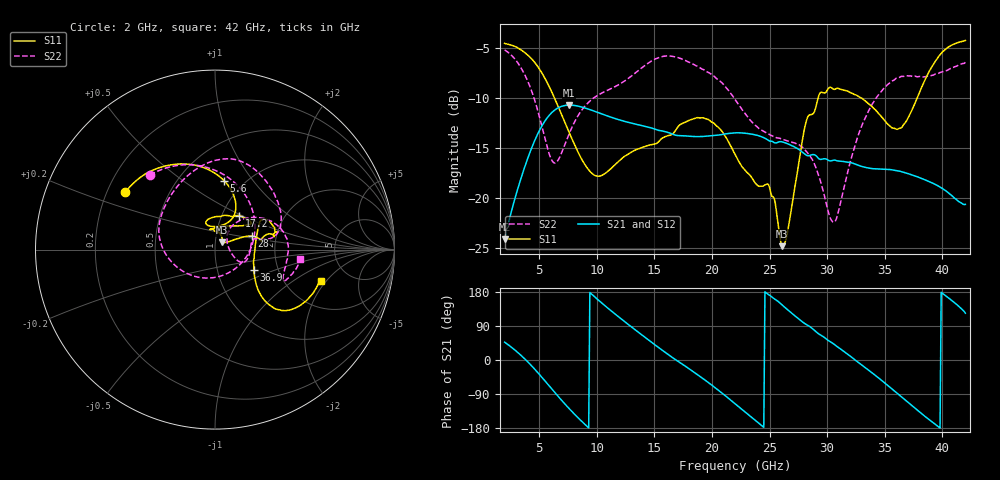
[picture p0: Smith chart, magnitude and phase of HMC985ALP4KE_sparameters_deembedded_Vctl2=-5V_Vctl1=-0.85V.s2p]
!s2p File: Measurements: S11, S21, S12, S22
# GHz S dB R 50.0
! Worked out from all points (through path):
!   401 points, 2 GHz to 42 GHz, reference 50 ohm
!   highest |S21| = -10.71 dB at 7.6 GHz (marker M1); lowest = -24.2 dB at 2 GHz (marker M2)
!   lowest |S11| = -24.9 dB at 26.1 GHz (marker M3), VSWR 1.12, Z = 54 + j4.44 ohm
!   |S11| at or under -10 dB: 6.33 GHz to 29.21 GHz (22.88 GHz wide, 129 % of centre); 32.97 GHz to 37.81 GHz (4.841 GHz wide, 13.7 % of centre)
!   |S22| runs from -22.4 to -5.2 dB; largest |S21 - S12| = 0.0003
!   S11 on the Smith chart (normalised r, x): 2 GHz: 0.27, +0.27; 5.6 GHz: 0.81, +0.73; 17.2 GHz: 1.21, +0.48; 28 GHz: 1.49, +0.24; 36.9 GHz: 1.50, -0.36; 42 GHz: 3.13, -1.75
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2  -4.52 147.5  -24.16 47.1  -24.17 47.1  -5.17 131.1
3.6  -5.31 120.9  -17.42 7.2  -17.42 7.2  -7.34 86.2
4.7  -6.56 100.0  -14.03 -27.1  -14.04 -27.1  -10.54 44.5
5.6  -8.24 82.5  -12.14 -58.6  -12.14 -58.6  -14.50 -5.9
6.4  -10.19 69.5  -11.16 -87.2  -11.17 -87.2  -16.51 -69.7
7.6  -13.45 60.7  -10.71 -128.1  -10.72 -128.2  -13.58 -142.4
8.7  -16.15 67.4  -10.90 -162.0  -10.90 -162.0  -11.20 -174.6
12  -16.25 109.1  -12.20 111.3  -12.21 111.4  -8.60 137.7
15.4  -14.34 78.2  -13.25 32.2  -13.25 32.2  -5.94 86.1
17.2  -12.69 54.5  -13.77 -6.1  -13.78 -6.1  -6.00 64.8
19.7  -12.16 35.7  -13.81 -59.8  -13.82 -59.8  -7.44 30.9
22  -15.62 52.9  -13.49 -115.2  -13.50 -115.2  -10.12 11.2
24.9  -18.66 98.6  -14.25 172.8  -14.26 172.9  -13.60 11.8
26.1  -24.85 45.8  -14.39 145.0  -14.40 145.0  -14.12 -1.3
28  -13.24 20.2  -15.58 97.4  -15.58 97.4  -15.10 -23.2
28.7  -11.63 10.6  -15.68 83.3  -15.68 83.4  -16.14 -26.1
30.6  -9.14 17.3  -16.22 41.5  -16.23 41.5  -22.45 19.5
33  -10.02 32.3  -16.86 -13.2  -16.86 -13.1  -12.79 47.5
35.4  -12.75 9.9  -17.17 -70.7  -17.17 -70.7  -8.52 20.5
36.9  -12.27 -27.7  -17.53 -108.9  -17.54 -108.9  -7.76 2.6
39.6  -5.97 -42.4  -18.79 -174.8  -18.79 -174.8  -7.56 -24.1
42  -4.23 -16.4  -20.66 123.4  -20.67 123.5  -6.42 -6.2
